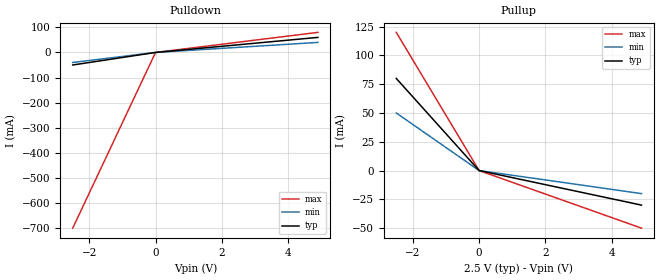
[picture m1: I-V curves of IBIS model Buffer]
|********************* IBIS GOLDEN PARSER BUG REPORT FORM *********************
|INSTRUCTIONS
|To report a bug in the IBIS golden parser.  Please fill out the top part
|of the following form and send the complete form to ibischk-bug@vhdl.org.
|A list of reported bugs will be maintained on vhdl.org.
|PARSER VERSION NUMBER:
|3.2.7
|PLATFORM (SPARC, HP700, PC, etc.):
|All
|OS AND VERSION:
|All
|REPORTED BY:
|Lance Wang (Cadence Design Systems. Inc.)
|DATE:
|7/20/2001
|DESCRIPTION OF BUG:
|Wrong line number of error for missing R,L C_pkg parameter(s).
|Error message is:
|ERROR (line  24) - Required sub-parameter L_pkg not found.
|But line number should be 12.
||INSERT IBIS FILE DEMONSTRATING THE BUG:
[IBIS Ver]   2.1
[File name]   bug58.ibs
[File Rev]   1.0
[Date]   July 23, 2001
[Component]   Component
[Manufacturer]  Generic
[Package]
|   typ   min   max
R_pkg   0.0000   0.0000   0.0000
|L_pkg   3.0nH   2nH   4nH
C_pkg   0.5pF   0.13pF   0.7pF
[Pin] signal_name   model_name   R_Pin   L_Pin   C_Pin
1   GND   GND   0.0000   5.000nH  0.400pF
2   Out   Buffer   0.0000   4.00nH   0.400pF
| Models and submodels in the file (1): Buffer (3-state)
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|   Buffer
[Model]   Buffer
Model_type   3-state
Vmeas = 1.25V
Rref = 1M
Vref = 0
| variable   typ   min   max
C_comp   2.0pF   NA   NA
[Temperature Range]   40.0   30   85.0
[Voltage range]   2.5V   2.3V   2.7V
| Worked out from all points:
|   slope of the pulldown table from 0 to 0.375 V, typ, clamps not added: 81.7 ohm
|   slope of the pullup table from 0 to 0.375 V, typ, clamps not added: 163 ohm
[Pullup]
|   Voltage   I(typ)   I(min)   I(max)
-2.5V     80mA       50mA       120mA
0V        0A         0A         0A
4.9V      -30mA      -20mA      -50mA
[Pulldown]
|   Voltage   I(typ)   I(min)   I(max)
-2.5V     -50mA      -40mA      -700mA
0V        0A         0A         0A
4.9V      60mA       40mA       80mA
[ramp]
| variable   typ   min   max
dV/dt_r   1/500p   .7/700p   1.13/500p
dV/dt_f   1/500p   .7/700p   1.1/300p
